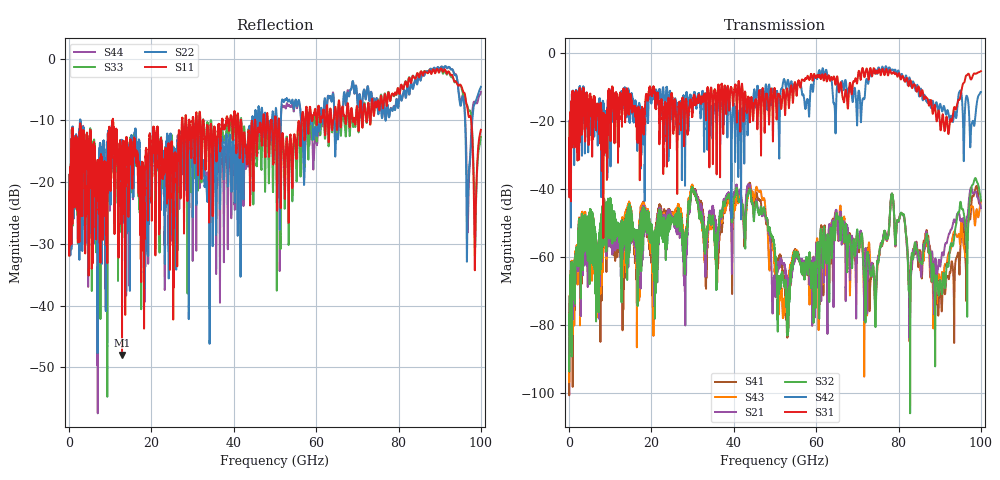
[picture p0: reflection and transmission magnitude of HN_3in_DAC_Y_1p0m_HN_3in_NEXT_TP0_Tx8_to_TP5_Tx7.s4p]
# GHz S RI R 45
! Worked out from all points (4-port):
!   4000 points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, 25 MHz to 100 GHz, reference 45 ohm
!   strongest paths, dB at 25 MHz, 25.02 GHz, 50.02 GHz, 75.03 GHz, 100 GHz:
!     S31: -38.9, -12.8, -11.0, -5.9, -5.4
!     S42: -38.9, -15.9, -12.9, -4.7, -11.5
!     S32: -89.2, -48.5, -58.5, -61.6, -43.4
!     S21: -88.7, -48.7, -66.3, -60.3, -45.6
!     S43: -87.2, -47.8, -66.7, -60.4, -43.5
!     S41: -88.2, -47.2, -60.2, -61.6, -43.4
!   lowest |S11| = -48.0 dB at 12.88 GHz (marker M1), VSWR 1.01, Z = 45 + j0.358 ohm
!   |S11| at or under -10 dB: start of sweep to 10.57 GHz; 10.66 GHz to 27.41 GHz (16.75 GHz wide, 88 % of centre); 51.03 GHz to 56.49 GHz (5.454 GHz wide, 10.1 % of centre)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
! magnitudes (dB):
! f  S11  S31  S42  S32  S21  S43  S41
! 25 MHz  -24.3  -38.9  -38.9  -89.2  -88.7  -87.2  -88.2
! 12.88 GHz  -48.0  -17.8  -11.6  -49.3  -50.3  -48.8  -49.2
! 45.85 GHz  -11.8  -18.0  -10.2  -46.2  -45.5  -40.5  -42.9
! 52.3 GHz  -19.0  -13.7  -7.9  -68.4  -62.7  -73.2  -67.9
! 78.42 GHz  -5.7  -6.1  -4.9  -41.3  -41.4  -41.4  -41.3
! 90.08 GHz  -1.8  -21.1  -15.0  -66.6  -62.7  -68.1  -67.9
! 100 GHz  -11.5  -5.4  -11.5  -43.4  -45.6  -43.5  -43.4
